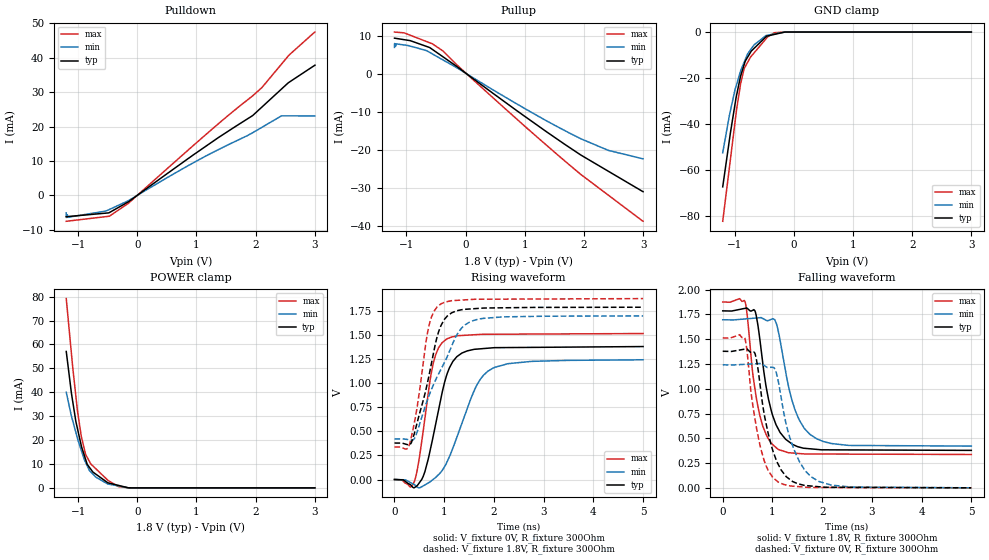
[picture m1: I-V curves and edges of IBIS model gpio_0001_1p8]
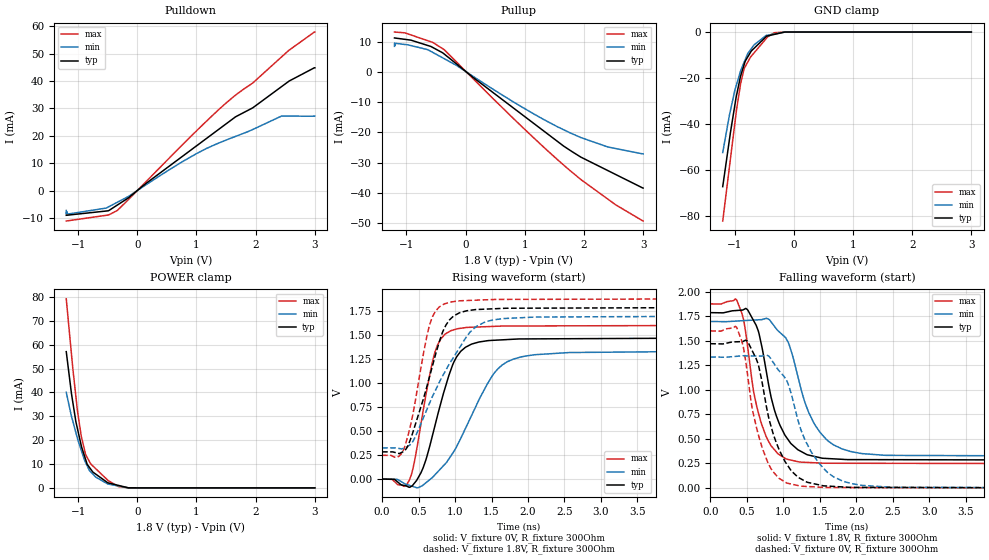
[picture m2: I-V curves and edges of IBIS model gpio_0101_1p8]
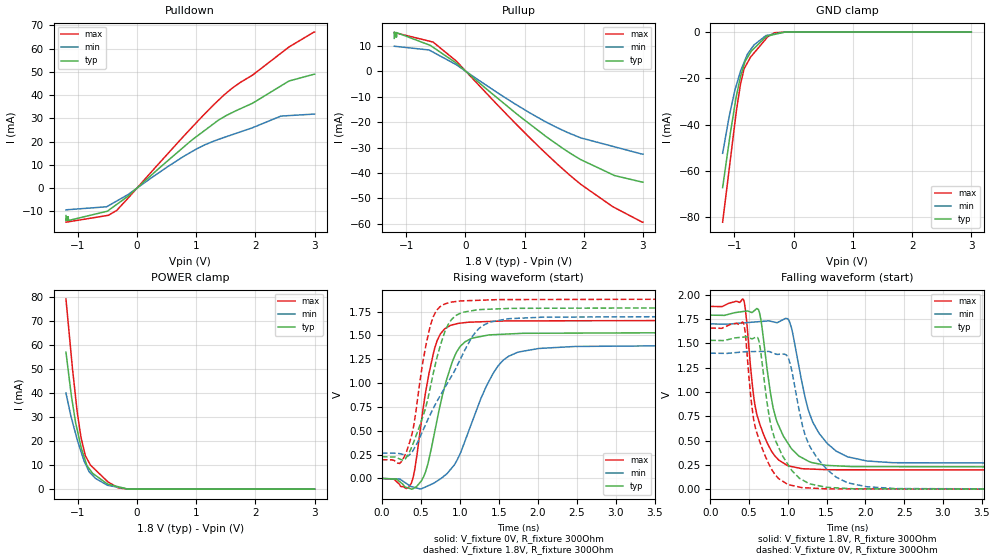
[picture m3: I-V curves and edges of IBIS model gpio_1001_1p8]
| Texas Instruments Incorporated
| DP83869
[IBIS Ver]   4.1
[File name]   dp83869.ibs
[File Rev]   1.5
[Date]   8/10/2018
[Source]
| Texas Instruments Incorporated.
| Analog-eLab Design Center, HPA
| 12500 TI Blvd
| Dallas, TX -75243
[Notes]   Revision History:
| Rev 1.5: 8/10/2018
| - Updated the gpio models for 1.8V, 2.5V and 3.3V
| Rev 1.4: 06/15/2018
| - Updated the models gpio_0110_1p8, gpio_1000_1p8, gpio_1110_1p8 and
|   gpio_1111_1p8 for 1.8V
| Rev 1.3: 06/11/2018
| - Included the model gpio_1111_1p8 for 1.8V
| Rev 1.2: 06/08/2018
| - Included the models gpio_0110_1p8, gpio_1000_1p8, gpio_1110_1p8 for 1.8V
| Rev 1.1: 04/13/2018
| - Included gpio and gpi models for 1.8V and 2.5V cases
| Rev 1.0: 04/04/2018
| - Initial version of the model.
| - Model generated from simulations in SPECTRE.
| - Model matched to SPICE simulation.
| - C_comp although listed in numerical order of value are
|   obtained from varying PVT conditions. For PVT conditions for
|   each specific value refer the buffer description under
|   respective [Model]. IBIS model user is responsible for using
|   appropriate C_comp to simulate for Signal Integrity.
| - Notes regarding non-monotonicity of various models
|   have been reviewed and considered minor and can be ignored.
| - Model names with a trailing _1p8 contain the model for 1.8V operation.
|   Model names with a trailing _2p5 contain the model for 2.5V operation.
|   Model names with a trailing _3p3 contain the model for 3.3V operation.
[Disclaimer]
| This model is designed as an aid for customers of Texas Instruments.
| TI and its licensors and suppliers make no warranties, either expressed
| or implied, with respect to this  model, including the warranties of
| merchantability or fitness for a particular purpose. The model is
| provided solely on an "as is" basis. The entire risk as to its quality
| and performance is with the customer.
| This model is subject to change without notice. Texas Instruments
| Incorporated is not responsible for updating this model.
[Copyright]
(C) Copyright 2018 Texas Instruments Incorporated.All rights reserved.
|  Component DP83869 48-pin QFN Package
|  Part # DP83869
[Component]   DP83869
[Manufacturer]   TI
[Package]   |48 QFN Package
|   typ   min   max
R_pkg   0.067   0.027   0.083
L_pkg   0.937nH   0.593nH   1.143nH
C_pkg   0.144pF   0.126pF   0.200pF
[Pin]  signal_name   model_name   R_pin   L_pin   C_pin
1   TD_P_A   nc   NA   NA   NA
2   TD_M_A   nc   NA   NA   NA
3   VDDA2P5   power   NA   NA   NA
4   TD_P_B   nc   NA   NA   NA
5   TD_M_B   nc   NA   NA   NA
6   VDD1P0   power   NA   NA   NA
7   TD_P_C   nc   NA   NA   NA
8   TD_M_C   nc   NA   NA   NA
9   VDDA2P5   power   NA   NA   NA
10   TD_P_D   nc   NA   NA   NA
11   TD_M_D   nc   NA   NA   NA
12   RBIAS   nc   NA   NA   NA
13   VDDA1P8   power   NA   NA   NA
14   SOP   diff_out   NA   NA   NA
15   SON   diff_out   NA   NA   NA
16   SIP   diff_in   NA   NA   NA
17   SIN   diff_in   NA   NA   NA
18   VDDIO   power   NA   NA   NA
19   XO   gpio   NA   NA   NA
20   XI   gpi   NA   NA   NA
21   JTAG_CLK   gpi   NA   NA   NA
22   JTAG_TDO/GPIO_1   gpio   NA   NA   NA
23   JTAG_TMS   gpi   NA   NA   NA
24   JTAG_TDI/SD   gpi   NA   NA   NA
25   TX_D3   gpi   NA   NA   NA
26   TX_D2   gpi   NA   NA   NA
27   TX_D1   gpi   NA   NA   NA
28   TX_D0   gpi   NA   NA   NA
29   GTX_CLK   gpi   NA   NA   NA
30   VDDIO   power   NA   NA   NA
31   VDD1P0   power   NA   NA   NA
32   RX_CLK   gpio   NA   NA   NA
33   RX_D0   gpio   NA   NA   NA
34   RX_D1   gpio   NA   NA   NA
35   RX_D2   gpio   NA   NA   NA
36   RX_D3   gpio   NA   NA   NA
37   TX_CTRL   gpi   NA   NA   NA
38   RX_CTRL   gpio   NA   NA   NA
39   VDD1P0   power   NA   NA   NA
40   CLK_OUT   gpio   NA   NA   NA
41   MDIO   gpio   NA   NA   NA
42   MDC   gpi   NA   NA   NA
43   RESET_N/POWERGOOD   gpi   NA   NA   NA
44   INT_N/PWDN_N   gpi   NA   NA   NA
45   LED_2/GPIO_0   gpio   NA   NA   NA
46   LED_1   gpio   NA   NA   NA
47   LED_0   gpio   NA   NA   NA
48   VDDA1P8   power   NA   NA   NA
[Diff Pin]   inv_pin   vdiff   tdelay_typ   tdelay_min   tdelay_max
14   15   NA   NA   NA   NA
16   17   0.15   NA   NA   NA
|   Model Selectors
[Model Selector]   gpio
gpio_0000_1p8   1.8V   Digital I/O
gpio_0001_1p8   1.8V   Digital I/O
gpio_0010_1p8   1.8V   Digital I/O
gpio_0011_1p8   1.8V   Digital I/O
gpio_0100_1p8   1.8V   Digital I/O
gpio_0101_1p8   1.8V   Digital I/O
gpio_0110_1p8   1.8V   Digital I/O
gpio_0111_1p8   1.8V   Digital I/O
gpio_1000_1p8   1.8V   Digital I/O
gpio_1001_1p8   1.8V   Digital I/O
gpio_1010_1p8   1.8V   Digital I/O
gpio_1011_1p8   1.8V   Digital I/O
gpio_1100_1p8   1.8V   Digital I/O
gpio_1101_1p8   1.8V   Digital I/O
gpio_1110_1p8   1.8V   Digital I/O
gpio_1111_1p8   1.8V   Digital I/O
gpio_0000_2p5   2.5V   Digital I/O
gpio_0001_2p5   2.5V   Digital I/O
gpio_0010_2p5   2.5V   Digital I/O
gpio_0011_2p5   2.5V   Digital I/O
gpio_0100_2p5   2.5V   Digital I/O
gpio_0101_2p5   2.5V   Digital I/O
gpio_0110_2p5   2.5V   Digital I/O
gpio_0111_2p5   2.5V   Digital I/O
gpio_1000_2p5   2.5V   Digital I/O
gpio_1001_2p5   2.5V   Digital I/O
gpio_1010_2p5   2.5V   Digital I/O
gpio_1011_2p5   2.5V   Digital I/O
gpio_1100_2p5   2.5V   Digital I/O
gpio_1101_2p5   2.5V   Digital I/O
gpio_1110_2p5   2.5V   Digital I/O
gpio_1111_2p5   2.5V   Digital I/O
gpio_0000_3p3   3.3V   Digital I/O
gpio_0001_3p3   3.3V   Digital I/O
gpio_0010_3p3   3.3V   Digital I/O
gpio_0011_3p3   3.3V   Digital I/O
gpio_0100_3p3   3.3V   Digital I/O
gpio_0101_3p3   3.3V   Digital I/O
gpio_0110_3p3   3.3V   Digital I/O
gpio_0111_3p3   3.3V   Digital I/O
gpio_1000_3p3   3.3V   Digital I/O
gpio_1001_3p3   3.3V   Digital I/O
gpio_1010_3p3   3.3V   Digital I/O
gpio_1011_3p3   3.3V   Digital I/O
gpio_1100_3p3   3.3V   Digital I/O
gpio_1101_3p3   3.3V   Digital I/O
gpio_1110_3p3   3.3V   Digital I/O
gpio_1111_3p3   3.3V   Digital I/O
[Model Selector]   gpi
gpi_1p8   1.8V   Digital Input
gpi_2p5   2.5V   Digital Input
gpi_3p3   3.3V   Digital Input
| Models and submodels in the file (53): diff_out (Output), diff_in (Input), gpio_0000_1p8 (I/O), gpio_0001_1p8 (I/O), gpio_0010_1p8 (I/O), gpio_0011_1p8 (I/O), gpio_0100_1p8 (I/O), gpio_0101_1p8 (I/O), gpio_0110_1p8 (I/O), gpio_0111_1p8 (I/O), gpio_1000_1p8 (I/O), gpio_1001_1p8 (I/O), gpio_1010_1p8 (I/O), gpio_1011_1p8 (I/O), gpio_1100_1p8 (I/O), gpio_1101_1p8 (I/O), gpio_1110_1p8 (I/O), gpio_1111_1p8 (I/O), gpio_0000_2p5 (I/O), gpio_0001_2p5 (I/O), gpio_0010_2p5 (I/O), gpio_0011_2p5 (I/O), gpio_0100_2p5 (I/O), gpio_0101_2p5 (I/O), gpio_0110_2p5 (I/O), gpio_0111_2p5 (I/O), gpio_1000_2p5 (I/O), gpio_1001_2p5 (I/O), gpio_1010_2p5 (I/O), gpio_1011_2p5 (I/O), gpio_1100_2p5 (I/O), gpio_1101_2p5 (I/O), gpio_1110_2p5 (I/O), gpio_1111_2p5 (I/O), gpio_0000_3p3 (I/O), gpio_0001_3p3 (I/O), gpio_0010_3p3 (I/O), gpio_0011_3p3 (I/O), gpio_0100_3p3 (I/O), gpio_0101_3p3 (I/O), gpio_0110_3p3 (I/O), gpio_0111_3p3 (I/O), gpio_1000_3p3 (I/O), gpio_1001_3p3 (I/O), gpio_1010_3p3 (I/O), gpio_1011_3p3 (I/O), gpio_1100_3p3 (I/O), gpio_1101_3p3 (I/O), gpio_1110_3p3 (I/O), gpio_1111_3p3 (I/O), gpi_1p8 (Input), gpi_2p5 (Input), gpi_3p3 (Input)
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|   gpio_0001_1p8 Model
[Model]   gpio_0001_1p8
Model_type   I/O
Polarity   Non-Inverting
Enable   Active-Low
Vinl = 0.344
Vinh = 1.204
Vmeas = 0.9
Vref = 0
Cref = 2pF
Rref = 100000
|   typ   min   max
C_comp   1.311pF   1.163pF   1.492pF
| Where Nom  PVT is Nominal Process, 1.8V,  27C
|   Fast PVT is Strong Process,  1.89V, -40C
|   Slow PVT is Weak Process,   1.71V, 125C
[Voltage Range]   1.8   1.71   1.89
|Junction Temperature
[Temperature Range]   27   125   -40
[Pullup Reference]   1.8   1.71   1.89
[Pulldown Reference]   -0   -0   0
[Power Clamp Reference]   1.8   1.71   1.89
[GND Clamp Reference]   0   0   0
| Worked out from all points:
|   slope of the pulldown table from 0 to 0.27 V, typ, clamps not added: 79.7 ohm
|   slope of the pullup table from 0 to 0.27 V, typ, clamps not added: 86.9 ohm
|   GND clamp passes 1 mA (typ) near -0.32 V on its own axis
|   POWER clamp passes 1 mA (typ) near -0.31 V on its own axis
|   falling waveform, V_fixture 1.8V, R_fixture 300Ohm: 20-80 % time 310ps typ, 378ps min, 267ps max; typ from 1.79 V to 0.378 V
|   rising waveform, V_fixture 0V, R_fixture 300Ohm: 20-80 % time 357ps typ, 557ps min, 261ps max; typ from 0 V to 1.38 V
|   rising waveform, V_fixture 1.8V, R_fixture 300Ohm: 20-80 % time 380ps typ, 630ps min, 262ps max; typ from 0.378 V to 1.79 V
|   falling waveform, V_fixture 0V, R_fixture 300Ohm: 20-80 % time 344ps typ, 416ps min, 295ps max; typ from 1.38 V to 0 V
[Pulldown]
|   Voltage   I(typ)   I(min)   I(max)
-1.2V     -6.204mA   -5.101mA   -7.537mA
-1.2V     -6.204mA   -6.141mA   -7.536mA
-1.199V   -6.202mA   -6.44mA    -7.535mA
-1.181V   -6.174mA   -5.638mA   -7.498mA
-1.176V   -6.167mA   -6.405mA   -7.488mA
-472.2mV  -5.01mA    -4.115mA   -6.068mA
-149.9mV  -1.89mA    -1.554mA   -2.313mA
991.5mV   12.29mA    9.888mA    15.16mA
1.951V    23.21mA    18.21mA    28.95mA
2.105V    25.65mA    19.77mA    31.31mA
2.436V    30.9mA     23.11mA    38.14mA
3V        37.84mA    23.09mA    47.46mA
[GND Clamp]
|   Voltage   I(typ)   I(min)   I(max)
-1.2V     -67.24mA   -52.42mA   -82.2mA
-1.087V   -46.83mA   -36.17mA   -58.77mA
-994.8mV  -31.76mA   -25.29mA   -39.68mA
-964.8mV  -27.33mA   -22.68mA   -33.46mA
-896.2mV  -18.98mA   -16.75mA   -22.25mA
-837.6mV  -14.13mA   -13.08mA   -15.89mA
-780.2mV  -10.95mA   -9.503mA   -13.19mA
-671.3mV  -7.107mA   -5.595mA   -9.089mA
-441mV    -1.68mA    -1.369mA   -2.105mA
-326mV    -1.017mA   -830.4uA   -284.6uA
-149.9mV  -2.237uA   -4.563uA   -2.286uA
3V        0A         0A         0A
[Pullup]
|   Voltage   I(typ)   I(min)   I(max)
-1.2V     9.343mA    6.922mA    10.95mA
-1.2V     9.343mA    7.694mA    10.95mA
-1.199V   9.34mA     7.943mA    10.95mA
-1.181V   9.296mA    7.248mA    10.92mA
-1.177V   9.287mA    7.859mA    10.92mA
-972mV    8.785mA    7.422mA    10.34mA
-604.8mV  6.876mA    5.597mA    8.13mA
-381.1mV  4.45mA     3.633mA    5.984mA
697.4mV   -7.775mA   -6.376mA   -9.558mA
1.946V    -21.31mA   -17.04mA   -26.4mA
2.411V    -25.58mA   -20.11mA   -31.85mA
3V        -30.96mA   -22.31mA   -38.73mA
[POWER Clamp]
|   Voltage   I(typ)   I(min)   I(max)
-1.2V     57.06mA    40.03mA    79.18mA
-1.112V   39.47mA    29.99mA    56.01mA
-1.038V   27.78mA    23.2mA     38.37mA
-1.012V   24.91mA    20.83mA    32.48mA
-946.6mV  17.69mA    15.73mA    21.61mA
-872.5mV  11.87mA    10.62mA    13.91mA
-845.3mV  9.809mA    9.184mA    12.68mA
-786mV    7.816mA    6.663mA    10.01mA
-492.1mV  2.077mA    1.587mA    3.051mA
-321.5mV  1.043mA    800uA      552.2uA
-149.9mV  3.276uA    7.968uA    3.523uA
3V        0A         0A         0A
[Ramp]
R_load = 300
|   typ   min   max
dV/dt_r   0.826936/3.56333e-10   0.744434/5.5534e-10   0.907942/2.59746e-10
dV/dt_f   0.844795/3.08178e-10   0.764979/3.75736e-10   0.923332/2.65255e-10
[Falling Waveform]
V_fixture = 1.8V
V_fixture_min = 1.71V
V_fixture_max = 1.89V
R_fixture = 300Ohm
C_fixture = 0F
|   Time   V(typ)   V(min)   V(max)
0s        1.786V     1.696V     1.875V
447.7ps   1.812V     1.704V     1.882V
646.9ps   1.788V     1.713V     1.003V
750.2ps   1.485V     1.717V     722.6mV
920.2ps   895.1mV    1.689V     494.1mV
1.104ns   606.6mV    1.611V     392.4mV
1.334ns   464.6mV    998.3mV    354.3mV
1.449ns   428.5mV    794.8mV    349.8mV
1.892ns   388mV      494.3mV    341.3mV
5ns       378.1mV    421.3mV    336.6mV
[Rising Waveform]
V_fixture = 0V
V_fixture_min = 0V
V_fixture_max = 0V
R_fixture = 300Ohm
C_fixture = 0F
|   Time   V(typ)   V(min)   V(max)
0s        156.4uV    376.3uV    113.3uV
316.7ps   -52.13mV   -29.83mV   -79mV
403ps     -83.36mV   -54.33mV   -17.55mV
578.9ps   34.24mV    -65.64mV   508.3mV
772.5ps   433.8mV    -1.038mV   1.188V
1.041ns   1.069V     165.8mV    1.454V
1.255ns   1.274V     439mV      1.488V
1.643ns   1.351V     965.8mV    1.502V
1.983ns   1.366V     1.155V     1.506V
5ns       1.378V     1.241V     1.513V
[Rising Waveform]
V_fixture = 1.8V
V_fixture_min = 1.71V
V_fixture_max = 1.89V
R_fixture = 300Ohm
C_fixture = 0F
|   Time   V(typ)   V(min)   V(max)
0s        378.1mV    421.3mV    336.6mV
296.6ps   359.1mV    411.8mV    356.7mV
430.2ps   537.8mV    456.3mV    674.3mV
688.6ps   1.064V     860.8mV    1.584V
790.6ps   1.326V     989.5mV    1.74V
931.4ps   1.591V     1.139V     1.82V
1.063ns   1.695V     1.277V     1.845V
1.285ns   1.753V     1.526V     1.858V
1.638ns   1.772V     1.656V     1.869V
5ns       1.786V     1.696V     1.875V
[Falling Waveform]
|Gnd
V_fixture = 0V
V_fixture_min = 0V
V_fixture_max = 0V
R_fixture = 300Ohm
C_fixture = 0F
|   Time   V(typ)   V(min)   V(max)
0s        1.378V     1.242V     1.513V
444.9ps   1.4V       1.246V     1.511V
642.4ps   1.363V     1.252V     714mV
833.9ps   745.8mV    1.235V     274.9mV
1.037ns   334.1mV    1.209V     91.71mV
1.114ns   239.9mV    1.085V     59.28mV
1.273ns   115.4mV    648.2mV    28.64mV
1.436ns   57.14mV    382.9mV    16.05mV
1.912ns   12.2mV     69.26mV    4.106mV
5ns       155.3uV    373uV      113.3uV
|   gpio_0101_1p8 Model
[Model]   gpio_0101_1p8
Model_type   I/O
Polarity   Non-Inverting
Enable   Active-Low
Vinl = 0.344
Vinh = 1.204
Vmeas = 0.9
Vref = 0
Cref = 2pF
Rref = 100000
|   typ   min   max
C_comp   1.311pF   1.163pF   1.492pF
| Where Nom  PVT is Nominal Process, 1.8V,  27C
|   Fast PVT is Strong Process,  1.89V, -40C
|   Slow PVT is Weak Process,   1.71V, 125C
[Voltage Range]   1.8   1.71   1.89
|Junction Temperature
[Temperature Range]   27   125   -40
[Pullup Reference]   1.8   1.71   1.89
[Pulldown Reference]   0   0   0
[Power Clamp Reference]   1.8   1.71   1.89
[GND Clamp Reference]   0   0   0
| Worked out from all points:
|   slope of the pulldown table from 0 to 0.27 V, typ, clamps not added: 59.1 ohm
|   slope of the pullup table from 0 to 0.27 V, typ, clamps not added: 65.4 ohm
|   GND clamp passes 1 mA (typ) near -0.32 V on its own axis
|   POWER clamp passes 1 mA (typ) near -0.31 V on its own axis
|   falling waveform, V_fixture 1.8V, R_fixture 300Ohm: 20-80 % time 298ps typ, 377ps min, 250ps max; typ from 1.79 V to 0.284 V
|   rising waveform, V_fixture 0V, R_fixture 300Ohm: 20-80 % time 325ps typ, 538ps min, 233ps max; typ from 0 V to 1.47 V
|   rising waveform, V_fixture 1.8V, R_fixture 300Ohm: 20-80 % time 347ps typ, 562ps min, 239ps max; typ from 0.284 V to 1.79 V
|   falling waveform, V_fixture 0V, R_fixture 300Ohm: 20-80 % time 324ps typ, 412ps min, 269ps max; typ from 1.47 V to 0 V
[Pulldown]
|   Voltage   I(typ)   I(min)   I(max)
-1.2V     -9.048mA   -7.268mA   -11.14mA
-1.2V     -9.048mA   -8.342mA   -11.14mA
-1.199V   -9.046mA   -8.607mA   -11.14mA
-1.191V   -9.027mA   -7.709mA   -11.11mA
-1.188V   -9.02mA    -8.59mA    -11.1mA
-1.151V   -8.934mA   -8.525mA   -10.99mA
-525.4mV  -7.489mA   -6.41mA    -9.052mA
-337.6mV  -5.312mA   -4.292mA   -7.297mA
799.1mV   13.08mA    11.01mA    17.51mA
1.326V    21.57mA    16.91mA    28.58mA
2.437V    37.97mA    27.22mA    48.82mA
3V        44.87mA    27.21mA    57.93mA
[GND Clamp]
|   Voltage   I(typ)   I(min)   I(max)
-1.2V     -67.24mA   -52.42mA   -82.2mA
-1.087V   -46.76mA   -36.12mA   -58.68mA
-994.6mV  -31.72mA   -25.26mA   -39.63mA
-965mV    -27.36mA   -22.71mA   -33.51mA
-896.4mV  -18.99mA   -16.77mA   -22.28mA
-837.8mV  -14.14mA   -13.09mA   -15.9mA
-780.4mV  -10.96mA   -9.511mA   -13.2mA
-671.9mV  -7.121mA   -5.61mA    -9.109mA
-441.2mV  -1.68mA    -1.372mA   -2.109mA
-326.4mV  -1.019mA   -832.9uA   -287uA
-149.7mV  -2.224uA   -4.058uA   -2.27uA
3V        0A         0A         0A
[Pullup]
|   Voltage   I(typ)   I(min)   I(max)
-1.2V     11.19mA    8.425mA    13.15mA
-1.2V     11.19mA    9.244mA    13.15mA
-1.199V   11.19mA    9.464mA    13.15mA
-1.191V   11.17mA    8.701mA    13.13mA
-1.188V   11.16mA    9.42mA     13.13mA
-971.2mV  10.6mA     8.913mA    12.52mA
-637.7mV  8.706mA    7.329mA    10.28mA
-360.8mV  5.901mA    4.363mA    7.328mA
1.087V    -16.04mA   -13.15mA   -20.58mA
1.75V     -25.68mA   -19.97mA   -32.3mA
2.407V    -32.6mA    -24.8mA    -42.03mA
3V        -38.36mA   -27.06mA   -49.22mA
[POWER Clamp]
|   Voltage   I(typ)   I(min)   I(max)
-1.2V     57.06mA    40.03mA    79.18mA
-1.112V   39.43mA    29.97mA    55.95mA
-1.038V   27.79mA    23.21mA    38.39mA
-1.012V   24.87mA    20.8mA     32.42mA
-946.7mV  17.7mA     15.75mA    21.64mA
-872.4mV  11.86mA    10.61mA    13.9mA
-845.5mV  9.821mA    9.196mA    12.69mA
-786.2mV  7.822mA    6.665mA    10.02mA
-492.1mV  2.079mA    1.585mA    3.05mA
-321.3mV  1.043mA    798.2uA    550.3uA
-149.7mV  3.252uA    7.488uA    3.484uA
3V        0A         0A         0A
[Ramp]
R_load = 300
|   typ   min   max
dV/dt_r   0.883044/3.23925e-10   0.801016/5.345e-10   0.961586/2.32071e-10
dV/dt_f   0.903375/2.94939e-10   0.824365/3.73865e-10   0.978868/2.47376e-10
[Falling Waveform]
V_fixture = 1.8V
V_fixture_min = 1.71V
V_fixture_max = 1.89V
R_fixture = 300Ohm
C_fixture = 0F
|   Time   V(typ)   V(min)   V(max)
0s        1.789V     1.699V     1.879V
362.9ps   1.811V     1.703V     1.915V
516.4ps   1.812V     1.71V      1.415V
597.8ps   1.702V     1.713V     965.9mV
704ps     1.45V      1.718V     648.5mV
876.3ps   802.6mV    1.652V     392.3mV
1.03ns    530.8mV    1.535V     298.9mV
1.418ns   322.5mV    664.1mV    256.6mV
1.807ns   291.4mV    397.2mV    251.1mV
5ns       283.6mV    325mV      247.5mV
[Rising Waveform]
V_fixture = 0V
V_fixture_min = 0V
V_fixture_max = 0V
R_fixture = 300Ohm
C_fixture = 0F
|   Time   V(typ)   V(min)   V(max)
0s        112.6uV    277.5uV    81.09uV
371.5ps   -85.82mV   -65.44mV   -15.42mV
445.5ps   -40.9mV    -83.17mV   188.5mV
564.8ps   121.2mV    -61.66mV   721.3mV
712.2ps   518.2mV    33.91mV    1.29V
941.9ps   1.136V     239.7mV    1.547V
1.144ns   1.375V     529.2mV    1.579V
1.511ns   1.446V     1.077V     1.592V
1.805ns   1.458V     1.252V     1.596V
5ns       1.472V     1.335V     1.603V
[Rising Waveform]
V_fixture = 1.8V
V_fixture_min = 1.71V
V_fixture_max = 1.89V
R_fixture = 300Ohm
C_fixture = 0F
|   Time   V(typ)   V(min)   V(max)
0s        283.6mV    325mV      247.5mV
200.8ps   272.5mV    322.1mV    224.2mV
298.9ps   290mV      322.3mV    312.6mV
414.6ps   468.8mV    381.8mV    645.2mV
646.3ps   1.055V     783.5mV    1.594V
852.7ps   1.57V      1.106V     1.826V
978.8ps   1.699V     1.269V     1.85V
1.205ns   1.759V     1.531V     1.863V
1.527ns   1.775V     1.66V      1.872V
5ns       1.789V     1.699V     1.879V
[Falling Waveform]
|Gnd
V_fixture = 0V
V_fixture_min = 0V
V_fixture_max = 0V
R_fixture = 300Ohm
C_fixture = 0F
|   Time   V(typ)   V(min)   V(max)
0s        1.472V     1.336V     1.603V
360.3ps   1.491V     1.343V     1.639V
510.5ps   1.495V     1.347V     1.156V
578.7ps   1.394V     1.347V     792.4mV
719.6ps   1.038V     1.347V     392.1mV
859.5ps   557.7mV    1.284V     165.5mV
1.042ns   249mV      1.101V     52.03mV
1.378ns   48.86mV    374.1mV    11.8mV
1.815ns   9.353mV    68.71mV    3.288mV
5ns       112.7uV    274.1uV    81.24uV
|   gpio_1001_1p8 Model
[Model]   gpio_1001_1p8
Model_type   I/O
Polarity   Non-Inverting
Enable   Active-Low
Vinl = 0.344
Vinh = 1.204
Vmeas = 0.9
Vref = 0
Cref = 2pF
Rref = 100000
|   typ   min   max
C_comp   1.311pF   1.163pF   1.492pF
| Where Nom  PVT is Nominal Process, 1.8V,  27C
|   Fast PVT is Strong Process,  1.89V, -40C
|   Slow PVT is Weak Process,   1.71V, 125C
[Voltage Range]   1.8   1.71   1.89
|Junction Temperature
[Temperature Range]   27   125   -40
[Pullup Reference]   1.8   1.71   1.89
[Pulldown Reference]   -0   0   -0
[Power Clamp Reference]   1.8   1.71   1.89
[GND Clamp Reference]   0   0   0
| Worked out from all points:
|   slope of the pulldown table from 0 to 0.27 V, typ, clamps not added: 43.7 ohm
|   slope of the pullup table from 0 to 0.27 V, typ, clamps not added: 50.1 ohm
|   GND clamp passes 1 mA (typ) near -0.32 V on its own axis
|   POWER clamp passes 1 mA (typ) near -0.31 V on its own axis
|   falling waveform, V_fixture 1.8V, R_fixture 300Ohm: 20-80 % time 251ps typ, 317ps min, 213ps max; typ from 1.79 V to 0.228 V
|   rising waveform, V_fixture 0V, R_fixture 300Ohm: 20-80 % time 272ps typ, 426ps min, 201ps max; typ from 0 V to 1.53 V
|   rising waveform, V_fixture 1.8V, R_fixture 300Ohm: 20-80 % time 304ps typ, 555ps min, 202ps max; typ from 0.228 V to 1.79 V
|   falling waveform, V_fixture 0V, R_fixture 300Ohm: 20-80 % time 281ps typ, 347ps min, 233ps max; typ from 1.53 V to 0 V
[Pulldown]
|   Voltage   I(typ)   I(min)   I(max)
-1.2V     -11.83mA   -9.367mA   -14.68mA
-1.199V   -14.01mA   -9.366mA   -14.68mA
-1.175V   -12.35mA   -9.319mA   -14.58mA
-1.172V   -13.95mA   -9.314mA   -14.57mA
-1.162V   -12.33mA   -9.294mA   -14.53mA
-1.147V   -13.89mA   -9.265mA   -14.46mA
-513.8mV  -10.03mA   -8.052mA   -11.85mA
-341.9mV  -7.016mA   -5.559mA   -9.593mA
788.5mV   17.67mA    13.64mA    22.32mA
1.471V    30.66mA    21.78mA    40.08mA
2.429V    43.93mA    30.96mA    58mA
3V        48.97mA    31.83mA    67.11mA
[GND Clamp]
|   Voltage   I(typ)   I(min)   I(max)
-1.2V     -67.24mA   -52.42mA   -82.2mA
-1.087V   -46.79mA   -36.15mA   -58.72mA
-994.6mV  -31.73mA   -25.27mA   -39.64mA
-964.5mV  -27.3mA    -22.66mA   -33.42mA
-896.4mV  -18.99mA   -16.77mA   -22.28mA
-837.5mV  -14.12mA   -13.07mA   -15.88mA
-780mV    -10.94mA   -9.494mA   -13.19mA
-671.1mV  -7.102mA   -5.591mA   -9.082mA
-440.8mV  -1.674mA   -1.365mA   -2.101mA
-325.9mV  -1.014mA   -828uA     -283.4uA
-149.4mV  -2.208uA   -4.034uA   -2.251uA
3V        0A         0A         0A
[Pullup]
|   Voltage   I(typ)   I(min)   I(max)
-1.2V     13.03mA    9.923mA    15.34mA
-1.2V     15.13mA    9.922mA    15.34mA
-1.199V   15.5mA     9.92mA     15.33mA
-1.175V   13.59mA    9.86mA     15.19mA
-1.172V   15.36mA    9.853mA    15.18mA
-1.162V   13.55mA    9.827mA    15.12mA
-1.159V   15.28mA    9.82mA     15.1mA
-543.4mV  9.486mA    7.57mA     11.54mA
1.082V    -20.64mA   -16.26mA   -26.02mA
1.809V    -32.79mA   -24.86mA   -41.77mA
2.521V    -41.04mA   -29.72mA   -53.68mA
3V        -43.62mA   -32.61mA   -59.41mA
[POWER Clamp]
|   Voltage   I(typ)   I(min)   I(max)
-1.2V     57.06mA    40.03mA    79.18mA
-1.112V   39.45mA    29.98mA    55.98mA
-1.038V   27.76mA    23.19mA    38.34mA
-1.012V   24.88mA    20.81mA    32.44mA
-946.5mV  17.68mA    15.73mA    21.6mA
-873.1mV  11.92mA    10.65mA    13.96mA
-845.2mV  9.805mA    9.18mA     12.69mA
-786.4mV  7.831mA    6.671mA    10.03mA
-492mV    2.075mA    1.583mA    3.048mA
-321.4mV  1.042mA    798.1uA    551.1uA
-149.4mV  3.224uA    7.439uA    3.455uA
3V        0A         0A         0A
[Ramp]
R_load = 300
|   typ   min   max
dV/dt_r   0.919087/2.72306e-10   0.839326/4.25675e-10   0.994788/2.00876e-10
dV/dt_f   0.937831/2.50292e-10   0.8608/3.13601e-10   1.01064/2.1292e-10
[Falling Waveform]
V_fixture = 1.8V
V_fixture_min = 1.71V
V_fixture_max = 1.89V
R_fixture = 300Ohm
C_fixture = 0F
|   Time   V(typ)   V(min)   V(max)
0s        1.791V     1.701V     1.881V
432.3ps   1.83V      1.712V     1.946V
562.9ps   1.834V     1.72V      942mV
620.9ps   1.849V     1.724V     717.2mV
810.8ps   838.6mV    1.722V     367.9mV
995.5ps   481.2mV    1.755V     243.8mV
1.049ns   416.1mV    1.658V     232.9mV
1.312ns   273.7mV    710.5mV    206.6mV
1.763ns   235mV      335.5mV    199.4mV
5ns       228.1mV    266.1mV    196.7mV
[Rising Waveform]
V_fixture = 0V
V_fixture_min = 0V
V_fixture_max = 0V
R_fixture = 300Ohm
C_fixture = 0F
|   Time   V(typ)   V(min)   V(max)
0s        88.65uV    221.9uV    62.8uV
377ps     -110.3mV   -84.54mV   -50.83mV
422.5ps   -96.5mV    -94.56mV   97.92mV
541ps     28.23mV    -96.05mV   798mV
664.3ps   435.1mV    -49.88mV   1.323V
878ps     1.159V     91.74mV    1.604V
1.067ns   1.433V     394.4mV    1.634V
1.418ns   1.507V     1.089V     1.647V
1.735ns   1.519V     1.321V     1.652V
5ns       1.532V     1.399V     1.658V
[Rising Waveform]
V_fixture = 1.8V
V_fixture_min = 1.71V
V_fixture_max = 1.89V
R_fixture = 300Ohm
C_fixture = 0F
|   Time   V(typ)   V(min)   V(max)
0s        228.1mV    266.1mV    196.7mV
228.4ps   204.7mV    260.1mV    157.8mV
314ps     221mV      238.8mV    275.5mV
407.7ps   380.3mV    304.9mV    550.6mV
523.3ps   642.9mV    496.8mV    1.208V
615.5ps   932.1mV    660.9mV    1.581V
806.4ps   1.534V     950.7mV    1.83V
1.162ns   1.76V      1.49V      1.866V
1.404ns   1.776V     1.643V     1.873V
5ns       1.791V     1.701V     1.881V
[Falling Waveform]
|Gnd
V_fixture = 0V
V_fixture_min = 0V
V_fixture_max = 0V
R_fixture = 300Ohm
C_fixture = 0F
|   Time   V(typ)   V(min)   V(max)
0s        1.532V     1.4V       1.658V
428.8ps   1.565V     1.413V     1.712V
454.3ps   1.567V     1.415V     1.586V
531.3ps   1.548V     1.416V     891.3mV
609.5ps   1.562V     1.417V     559.8mV
791.6ps   625.4mV    1.407V     204.8mV
995.5ps   263mV      1.363V     50.93mV
1.273ns   58.51mV    459.3mV    12.3mV
1.763ns   7.843mV    68.31mV    2.908mV
5ns       88.13uV    218.9uV    63.02uV
